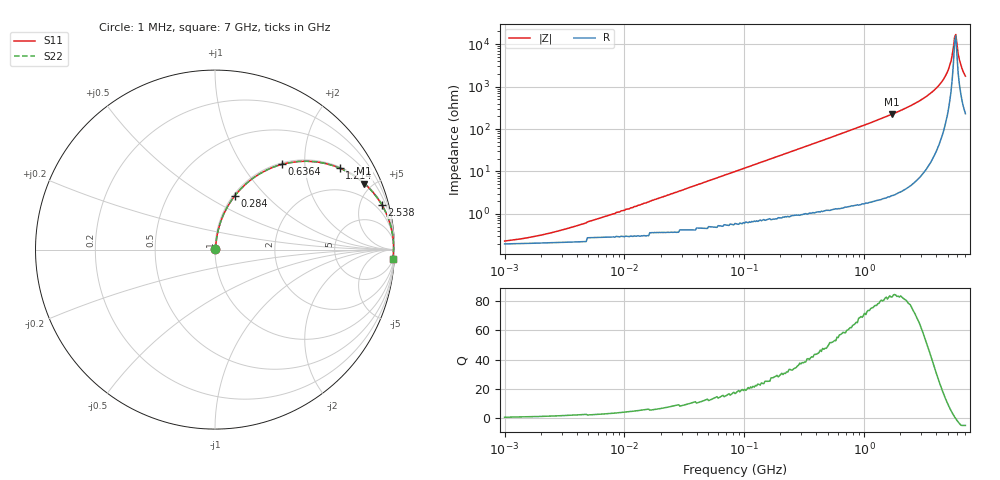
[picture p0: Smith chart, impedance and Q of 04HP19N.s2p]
# MHz S MA R 50
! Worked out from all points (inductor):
!   385 points, 1 MHz to 7 GHz, reference 50 ohm
!   read as one part in series: L = 19 nH near 7.263 MHz
!   highest Q = 83.6 at 1.715 GHz (marker M1), where L = 20.8 nH
!   self-resonance near 5.688 GHz
!   S11 on the Smith chart (normalised r, x): 1 MHz: 1.00, +0.00; 284 MHz: 1.02, +0.68; 636.4 MHz: 1.03, +1.54; 1.214 GHz: 1.04, +3.03; 2.538 GHz: 1.10, +7.51; 7 GHz: 6, -35
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1  0.002257 31.8  0.998 -0.1  0.998 -0.1  0.002257 31.8
1.952  0.003134 47.7  0.998 -0.1  0.998 -0.1  0.003134 47.7
4.374  0.005746 64.7  0.998 -0.3  0.998 -0.3  0.005746 64.7
19.575  0.024 80.1  0.996 -1.3  0.996 -1.3  0.024 80.1
85.617  0.101 80.9  0.989 -5.8  0.989 -5.8  0.101 80.9
283.957  0.319 69.8  0.939 -18.6  0.939 -18.6  0.319 69.8
365.931  0.398 65.2  0.908 -23.5  0.908 -23.5  0.398 65.2
636.381  0.605 51.8  0.786 -37.2  0.786 -37.2  0.605 51.8
1213.638  0.83 33.2  0.547 -56.1  0.547 -56.1  0.83 33.2
1637.803  0.901 25.1  0.424 -64.2  0.424 -64.2  0.901 25.1
1715.095  0.909 23.9  0.405 -65.4  0.405 -65.4  0.909 23.9
2538.13  0.963 14.9  0.256 -74.4  0.256 -74.4  0.963 14.9
3586.848  0.987 8.1  0.142 -80.5  0.142 -80.5  0.987 8.1
4622.31  0.994 3.7  0.065 -82.8  0.065 -82.8  0.994 3.7
4953.349  0.995 2.5  0.045 -81.9  0.045 -81.9  0.995 2.5
5308.095  0.995 1.4  0.025 -77.6  0.025 -77.6  0.995 1.4
5558.598  0.995 0.6  0.012 -64.8  0.012 -64.8  0.995 0.6
5688.248  0.995 0.3  0.006846 -39.9  0.006846 -39.9  0.995 0.3
5820.923  0.995 -0.1  0.005858 22.3  0.005858 22.3  0.995 -0.1
6095.627  0.994 -0.9  0.017 68.6  0.017 68.6  0.994 -0.9
6237.803  0.994 -1.3  0.023 73.5  0.023 73.5  0.994 -1.3
7000  0.991 -3.2  0.056 79.3  0.056 79.3  0.991 -3.2
